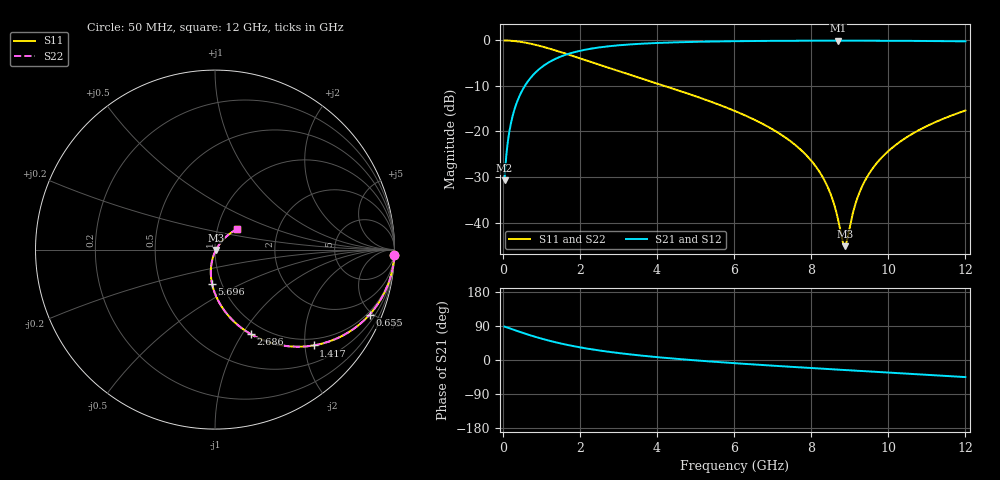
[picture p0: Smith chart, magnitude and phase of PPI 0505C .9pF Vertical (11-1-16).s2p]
# GHz S MA R 50
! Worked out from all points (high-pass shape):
!   1601 points, 50 MHz to 12 GHz, reference 50 ohm
!   highest |S21| = -0.05 dB at 8.699 GHz (marker M1); lowest = -30.8 dB at 50 MHz (marker M2)
!   |S21| within 3 dB of the highest: 1.667 GHz to end of sweep
!   lowest |S11| = -45.2 dB at 8.871 GHz (marker M3), VSWR 1.01, Z = 50.5 - j0.247 ohm
!   |S11| at or under -10 dB: 4.205 GHz to end of sweep
!   |S22| runs from -45.2 to 0.0 dB; largest |S21 - S12| = 0
!   S11 on the Smith chart (normalised r, x): 50 MHz: 1, -63; 655 MHz: 0.84, -4.81; 1.417 GHz: 0.85, -2.19; 2.686 GHz: 0.86, -1.09; 5.696 GHz: 0.90, -0.36; 12 GHz: 1.25, +0.30
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0.05  0.9996 -1.8  0.02896 88.2  0.02896 88.2  0.9996 -1.8
0.1620312  0.9956 -5.9  0.0935 84.1  0.0935 84.1  0.9956 -5.9
0.2665938  0.9882 -9.6  0.1528 80.4  0.1528 80.4  0.9882 -9.6
0.4309062  0.97 -15.4  0.2426 74.6  0.2426 74.6  0.97 -15.4
0.6549687  0.9342 -22.9  0.356 67.1  0.356 67.1  0.9342 -22.9
1.416781  0.7658 -44.2  0.6414 45.7  0.6414 45.7  0.7658 -44.2
2.044156  0.6279 -57.1  0.776 32.7  0.776 32.7  0.6279 -57.1
2.686469  0.5106 -67.2  0.857 22.6  0.857 22.6  0.5106 -67.2
4.038312  0.3334 -82.2  0.9391 7.3  0.9391 7.3  0.3334 -82.2
5.696375  0.1907 -94.9  0.9772 -6.2  0.9772 -6.2  0.1907 -94.9
6.025  0.1677 -97.0  0.9812 -8.5  0.9812 -8.5  0.1677 -97.0
7.227469  0.09201 -103.4  0.9905 -16.4  0.9905 -16.4  0.09201 -103.4
8.019156  0.04688 -105.0  0.9933 -21.3  0.9933 -21.3  0.04688 -105.0
8.429937  0.02451 -101.3  0.9939 -23.8  0.9939 -23.8  0.02451 -101.3
8.698813  0.01075 -85.1  0.994 -25.4  0.994 -25.4  0.01075 -85.1
8.810844  0.006352 -56.5  0.994 -26.1  0.994 -26.1  0.006352 -56.5
8.870594  0.005502 -26.4  0.9939 -26.4  0.9939 -26.4  0.005502 -26.4
9.146937  0.01591 41.2  0.9937 -28.1  0.9937 -28.1  0.01591 41.2
9.333656  0.02555 47.9  0.9934 -29.2  0.9934 -29.2  0.02555 47.9
10.01331  0.06158 51.1  0.9914 -33.2  0.9914 -33.2  0.06158 51.1
10.84981  0.1065 48.3  0.9872 -38.2  0.9872 -38.2  0.1065 48.3
12  0.1699 42.5  0.9777 -45.1  0.9777 -45.1  0.1699 42.5
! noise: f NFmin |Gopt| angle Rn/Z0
0.05  0.001231  0.9722  1.435  0.01005
1.372  0.005838  0.7709  6.647  0.005179
2.701  0.009176  0.7174  10.11  0.006372
4.031  0.01214  0.6864  13.67  0.007413
5.36  0.01494  0.6659  17.24  0.00839
6.682  0.01766  0.6521  20.75  0.009356
8.012  0.02041  0.6432  24.23  0.01037
9.341  0.02322  0.6382  27.64  0.01145
10.67  0.02616  0.6366  30.99  0.01264
12  0.02926  0.6381  34.26  0.01399
